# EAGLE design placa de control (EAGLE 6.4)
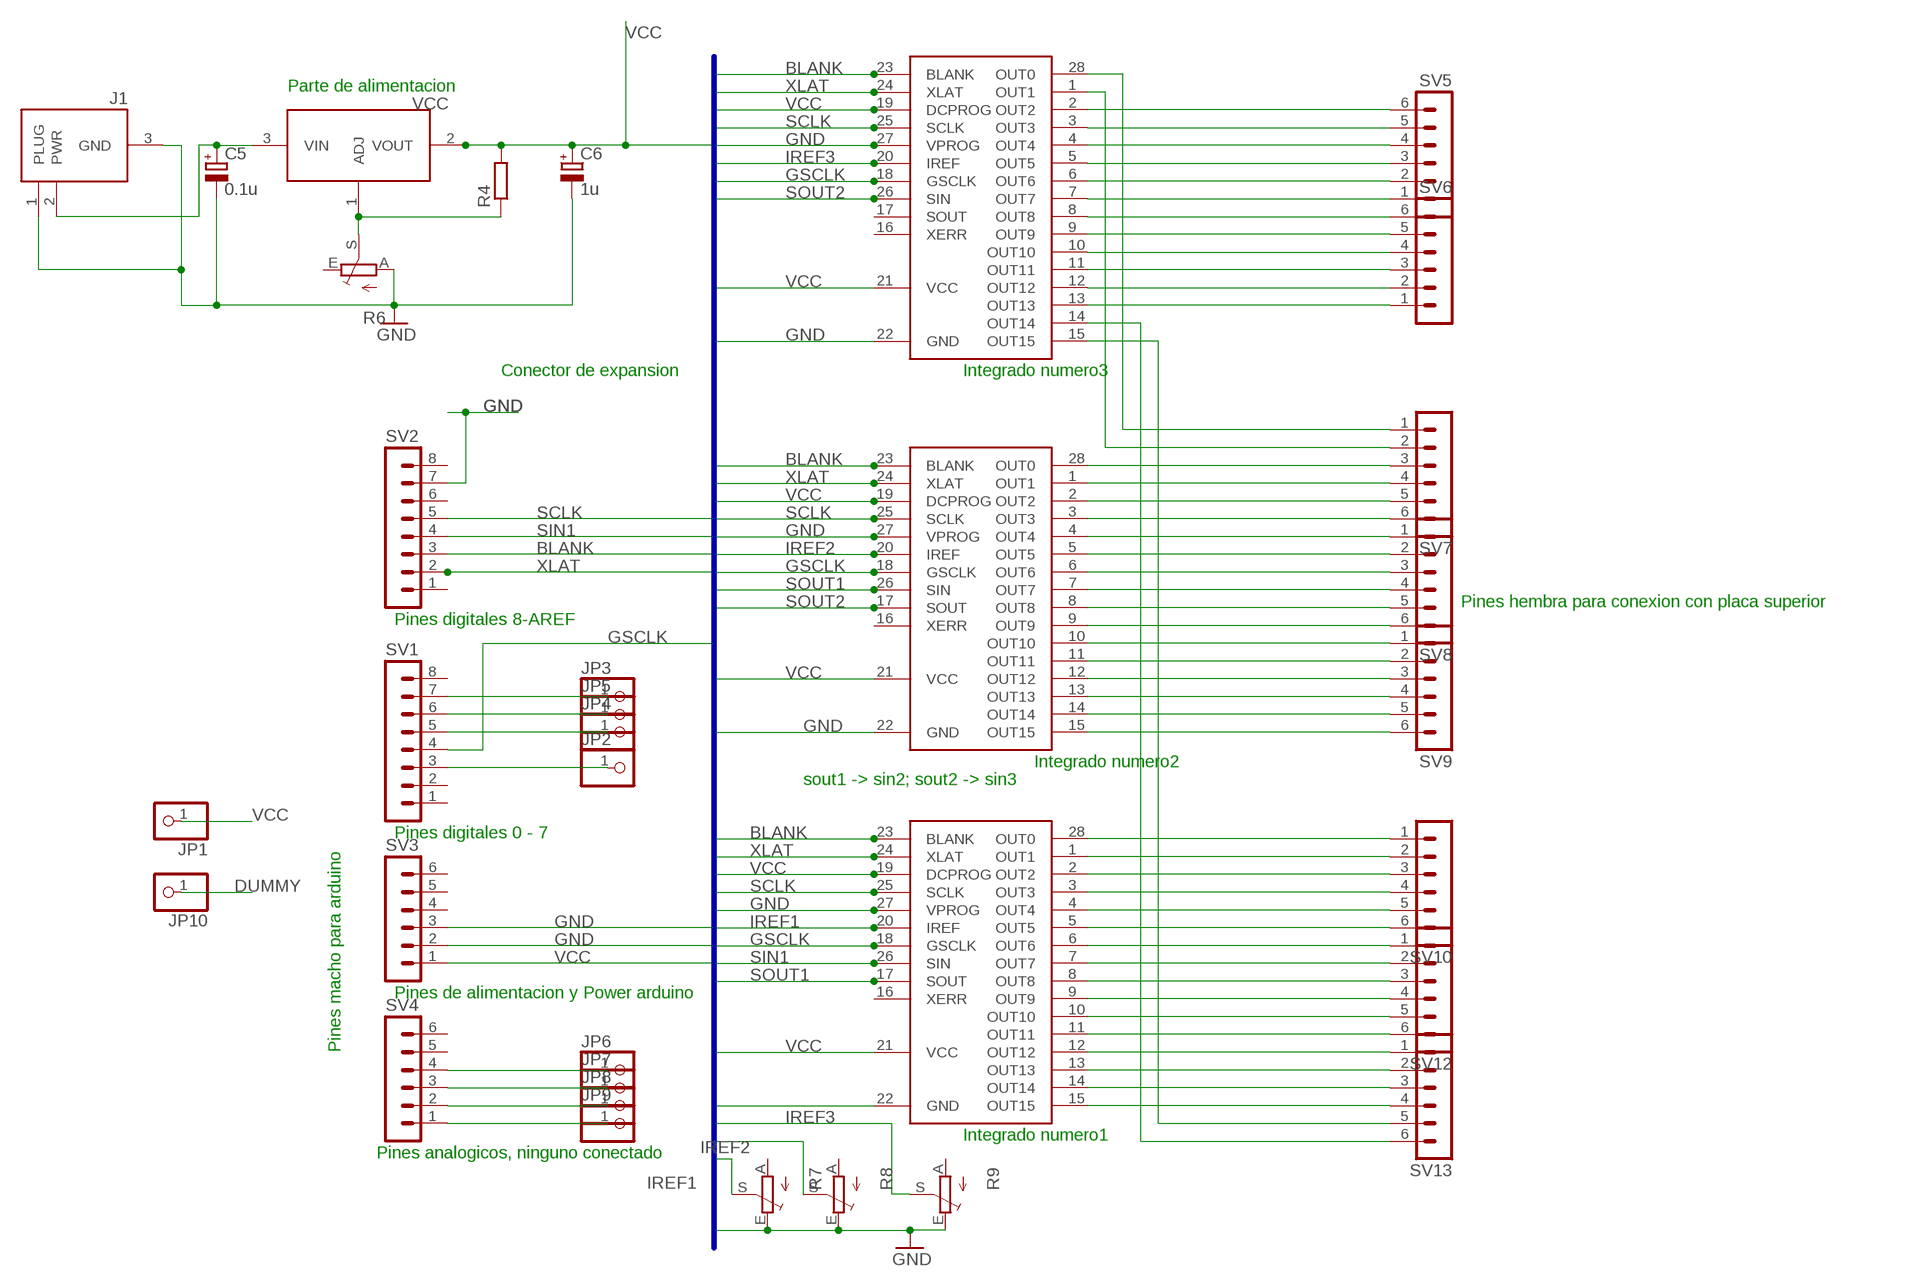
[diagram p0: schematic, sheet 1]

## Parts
C5  0.1u  CPOL-EUE2,5-6E  [E2,5-6E]
C6  1u  CPOL-EUE2,5-6E  [E2,5-6E]
J1  DCJACK-21MM  [DC-21MM]
JP1  PINHD-1X1  [1X01]
JP2  PINHD-1X1  [1X01]
JP3  PINHD-1X1  [1X01]
JP4  PINHD-1X1  [1X01]
JP5  PINHD-1X1  [1X01]
JP6  PINHD-1X1  [1X01]
JP7  PINHD-1X1  [1X01]
JP8  PINHD-1X1  [1X01]
JP9  PINHD-1X1  [1X01]
JP10  PINHD-1X1  [1X01]
R4  R-EU_0204/5  [0204/5]
R6  TRIM_EU-CA9V  [CA9V]
R7  TRIM_EU-CA9V  [CA9V]
R8  TRIM_EU-CA9V  [CA9V]
R9  TRIM_EU-CA9V  [CA9V]
SV1  MA08-1  [MA08-1]
SV2  MA08-1  [MA08-1]
SV3  MA06-1  [MA06-1]
SV4  MA06-1  [MA06-1]
SV5  MA06-1  [MA06-1]
SV6  MA06-1  [MA06-1]
SV7  MA06-1  [MA06-1]
SV8  MA06-1  [MA06-1]
SV9  MA06-1  [MA06-1]
SV10  MA06-1  [MA06-1]
SV12  MA06-1  [MA06-1]
SV13  MA06-1  [MA06-1]
U$1  TLC5940  [DIL28-3]
U$2  TLC5940  [DIL28-3]
U$3  TLC5940  [DIL28-3]
U$4  LM350T  [TO220]

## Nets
ADJ [Vcc]: R4.1 R6.S U$4.1(ADJ)
BLANK: SV2.3 U$1.23(BLANK) U$2.23(BLANK) U$3.23(BLANK)
DUMMY: JP10.1
GND [Vcc]: C5.- C6.- J1.1(PLUG) J1.3(GND) R6.A R7.E R8.E R9.E SV2.7 SV3.2 SV3.3 U$1.22(GND) U$1.27(VPROG) U$2.22(GND) U$2.27(VPROG) U$3.22(GND) U$3.27(VPROG)
GSCLK: SV1.4 U$1.18(GSCLK) U$2.18(GSCLK) U$3.18(GSCLK)
IREF1: R7.S U$2.20(IREF)
IREF2: R8.S U$1.20(IREF)
IREF3: R9.S U$3.20(IREF)
N$2: JP9.1 SV4.1
N$3 [Vcc]: C5.+ J1.2(PWR) U$4.3(VIN)
N$4: JP8.1 SV4.2
N$5: JP7.1 SV4.3
N$6: JP6.1 SV4.4
N$7: JP2.1 SV1.3
N$8: JP3.1 SV1.7
N$9: JP4.1 SV1.5
N$10: JP5.1 SV1.6
N$11: SV10.1 U$2.28(OUT0)
N$12: SV10.2 U$2.1(OUT1)
N$13: SV10.3 U$2.2(OUT2)
N$14: SV10.4 U$2.3(OUT3)
N$15: SV10.5 U$2.4(OUT4)
N$16: SV10.6 U$2.5(OUT5)
N$17: SV12.1 U$2.6(OUT6)
N$18: SV12.2 U$2.7(OUT7)
N$19: SV12.3 U$2.8(OUT8)
N$20: SV12.4 U$2.9(OUT9)
N$21: SV12.5 U$2.10(OUT10)
N$22: SV12.6 U$2.11(OUT11)
N$23: SV13.1 U$2.12(OUT12)
N$24: SV13.2 U$2.13(OUT13)
N$25: SV13.3 U$2.14(OUT14)
N$26: SV13.4 U$2.15(OUT15)
N$27: SV13.5 U$3.15(OUT15)
N$28: SV13.6 U$3.14(OUT14)
N$29: SV9.1 U$1.10(OUT10)
N$30: SV9.2 U$1.11(OUT11)
N$31: SV9.3 U$1.12(OUT12)
N$32: SV9.4 U$1.13(OUT13)
N$33: SV9.5 U$1.14(OUT14)
N$34: SV9.6 U$1.15(OUT15)
N$35: SV8.1 U$1.4(OUT4)
N$36: SV8.2 U$1.5(OUT5)
N$37: SV8.3 U$1.6(OUT6)
N$38: SV8.4 U$1.7(OUT7)
N$39: SV8.5 U$1.8(OUT8)
N$40: SV8.6 U$1.9(OUT9)
N$41: SV7.3 U$1.28(OUT0)
N$42: SV7.4 U$1.1(OUT1)
N$43: SV7.5 U$1.2(OUT2)
N$44: SV7.6 U$1.3(OUT3)
N$45: SV7.1 U$3.28(OUT0)
N$46: SV7.2 U$3.1(OUT1)
N$47: SV5.6 U$3.2(OUT2)
N$48: SV5.5 U$3.3(OUT3)
N$49: SV5.4 U$3.4(OUT4)
N$50: SV5.3 U$3.5(OUT5)
N$51: SV5.2 U$3.6(OUT6)
N$52: SV5.1 U$3.7(OUT7)
N$53: SV6.6 U$3.8(OUT8)
N$54: SV6.5 U$3.9(OUT9)
N$55: SV6.4 U$3.10(OUT10)
N$56: SV6.3 U$3.11(OUT11)
N$57: SV6.2 U$3.12(OUT12)
N$58: SV6.1 U$3.13(OUT13)
SCLK: SV2.5 U$1.25(SCLK) U$2.25(SCLK) U$3.25(SCLK)
SIN1: SV2.4 U$2.26(SIN)
SOUT1: U$1.26(SIN) U$2.17(SOUT)
SOUT2: U$1.17(SOUT) U$3.26(SIN)
VCC [Vcc]: C6.+ JP1.1 R4.2 SV3.1 U$1.19(DCPROG) U$1.21(VCC) U$2.19(DCPROG) U$2.21(VCC) U$3.19(DCPROG) U$3.21(VCC) U$4.2(VOUT)
XLAT: SV2.2 U$1.24(XLAT) U$2.24(XLAT) U$3.24(XLAT)
Unconnected: R6.E R7.A R8.A R9.A SV1.1 SV1.2 SV1.8 SV2.1 SV2.6 SV2.8 SV3.4 SV3.5 SV3.6 SV4.5 SV4.6 U$1.16(XERR) U$2.16(XERR) U$3.16(XERR) U$3.17(SOUT)

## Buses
VCC,GND,BLANK,SIN1,SOUT1,SOUT2,GSCLK,SCLK,XLAT,IREF1,IREF2,IREF3

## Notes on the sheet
- Parte de alimentacion
- Conector de expansion | Integrado numero3
- Pines hembra para conexion con placa superior
- Pines digitales 8-AREF
- Integrado numero2
- sout1 -> sin2; sout2 -> sin3
- Pines digitales 0 - 7
- Pines de alimentacion y Power arduino
- Pines macho para arduino
- Integrado numero1
- Pines analogicos, ninguno conectado

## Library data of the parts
C5 C6 = resistor:CPOL-EU: POLARIZED CAPACITOR, European symbol
J1 = powersupply:DCJACK: 2.1mm DC Power Jack Mouser Part No. 163-5004
JP1-JP10 = pinhead:PINHD-1X1: PIN HEADER
R4 = resistor:R-EU_: RESISTOR, European symbol
R6-R9 = pot:TRIM_EU-: POTENTIOMETER
SV1 SV2 = con-lstb:MA08-1: PIN HEADER; OC_FARNELL: unknown; OC_NEWARK: unknown
SV3-SV10 SV12 SV13 = con-lstb:MA06-1: PIN HEADER; OC_FARNELL: unknown; OC_NEWARK: unknown
U$1-U$3 = tlc5940:TLC5940
U$4 = tlc5940:LM350T

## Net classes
0 Normal: width 0.559 mm, drill 0.559 mm, clearance 0.559 mm
1 Vcc: width 0.762 mm, drill 0.762 mm, clearance 0.762 mm to class 0, clearance 0.762 mm

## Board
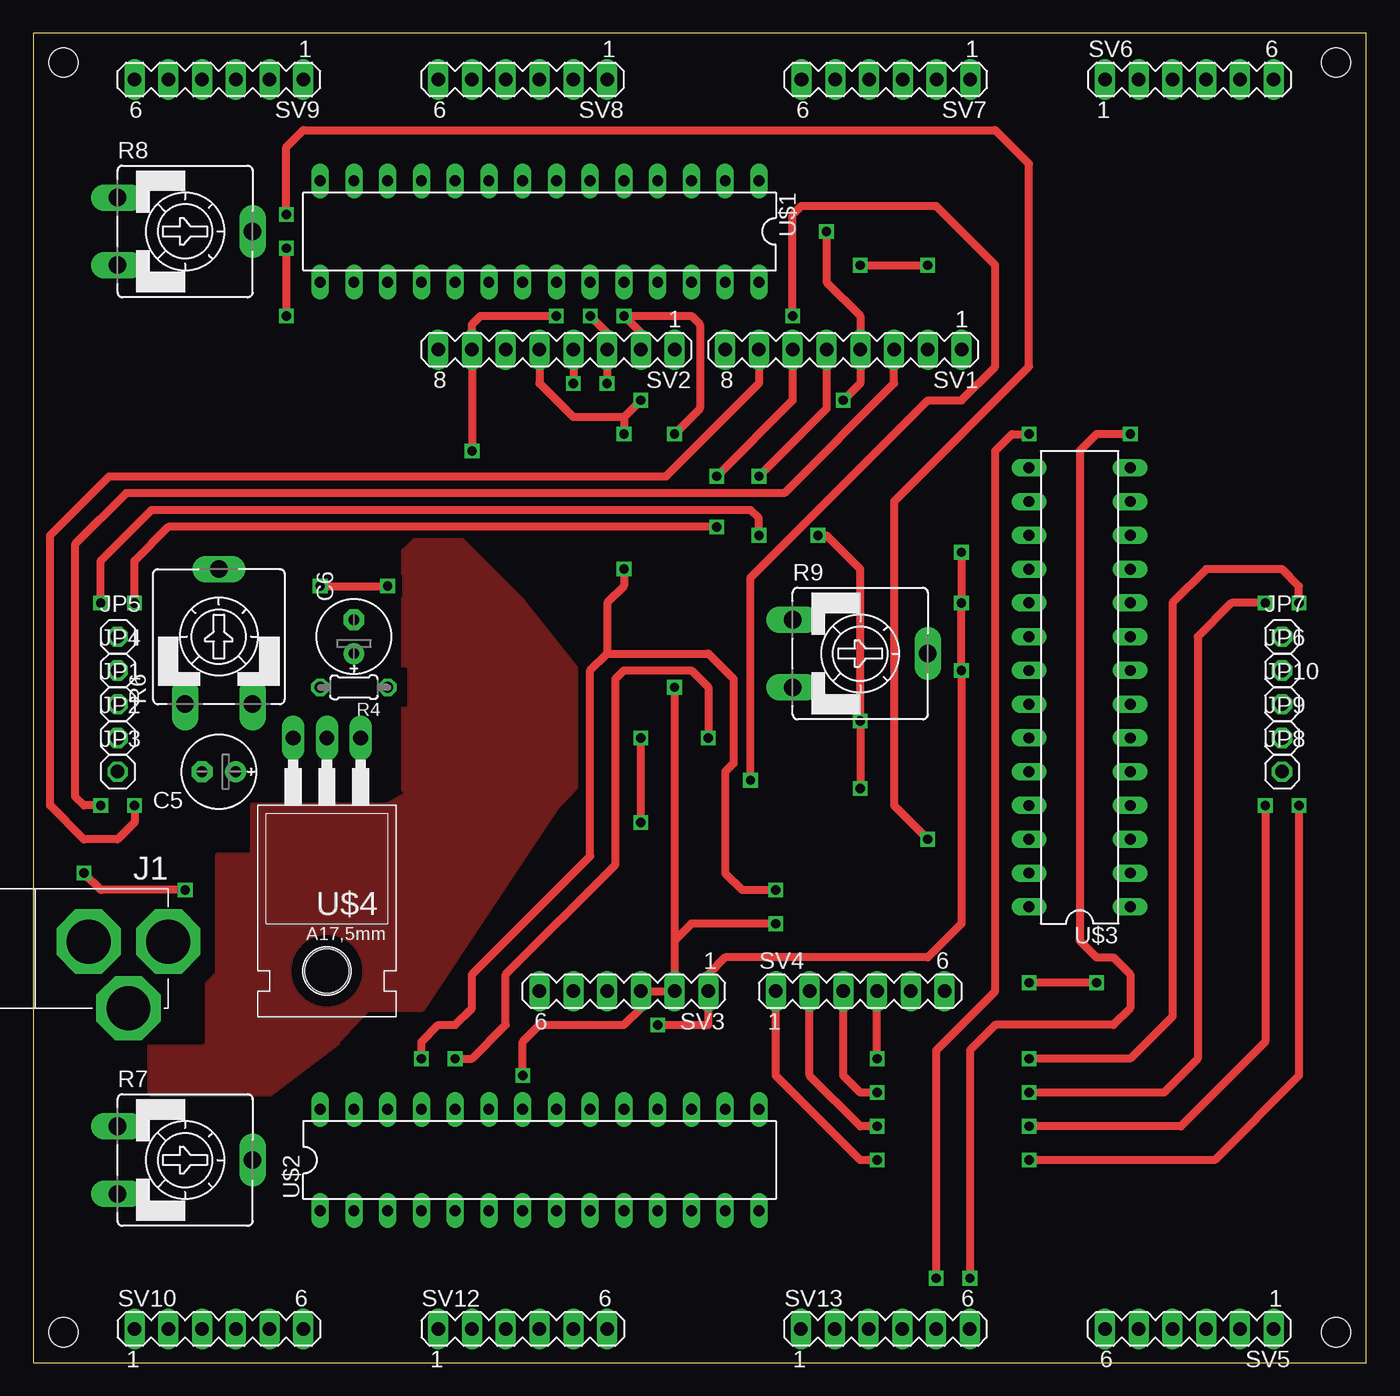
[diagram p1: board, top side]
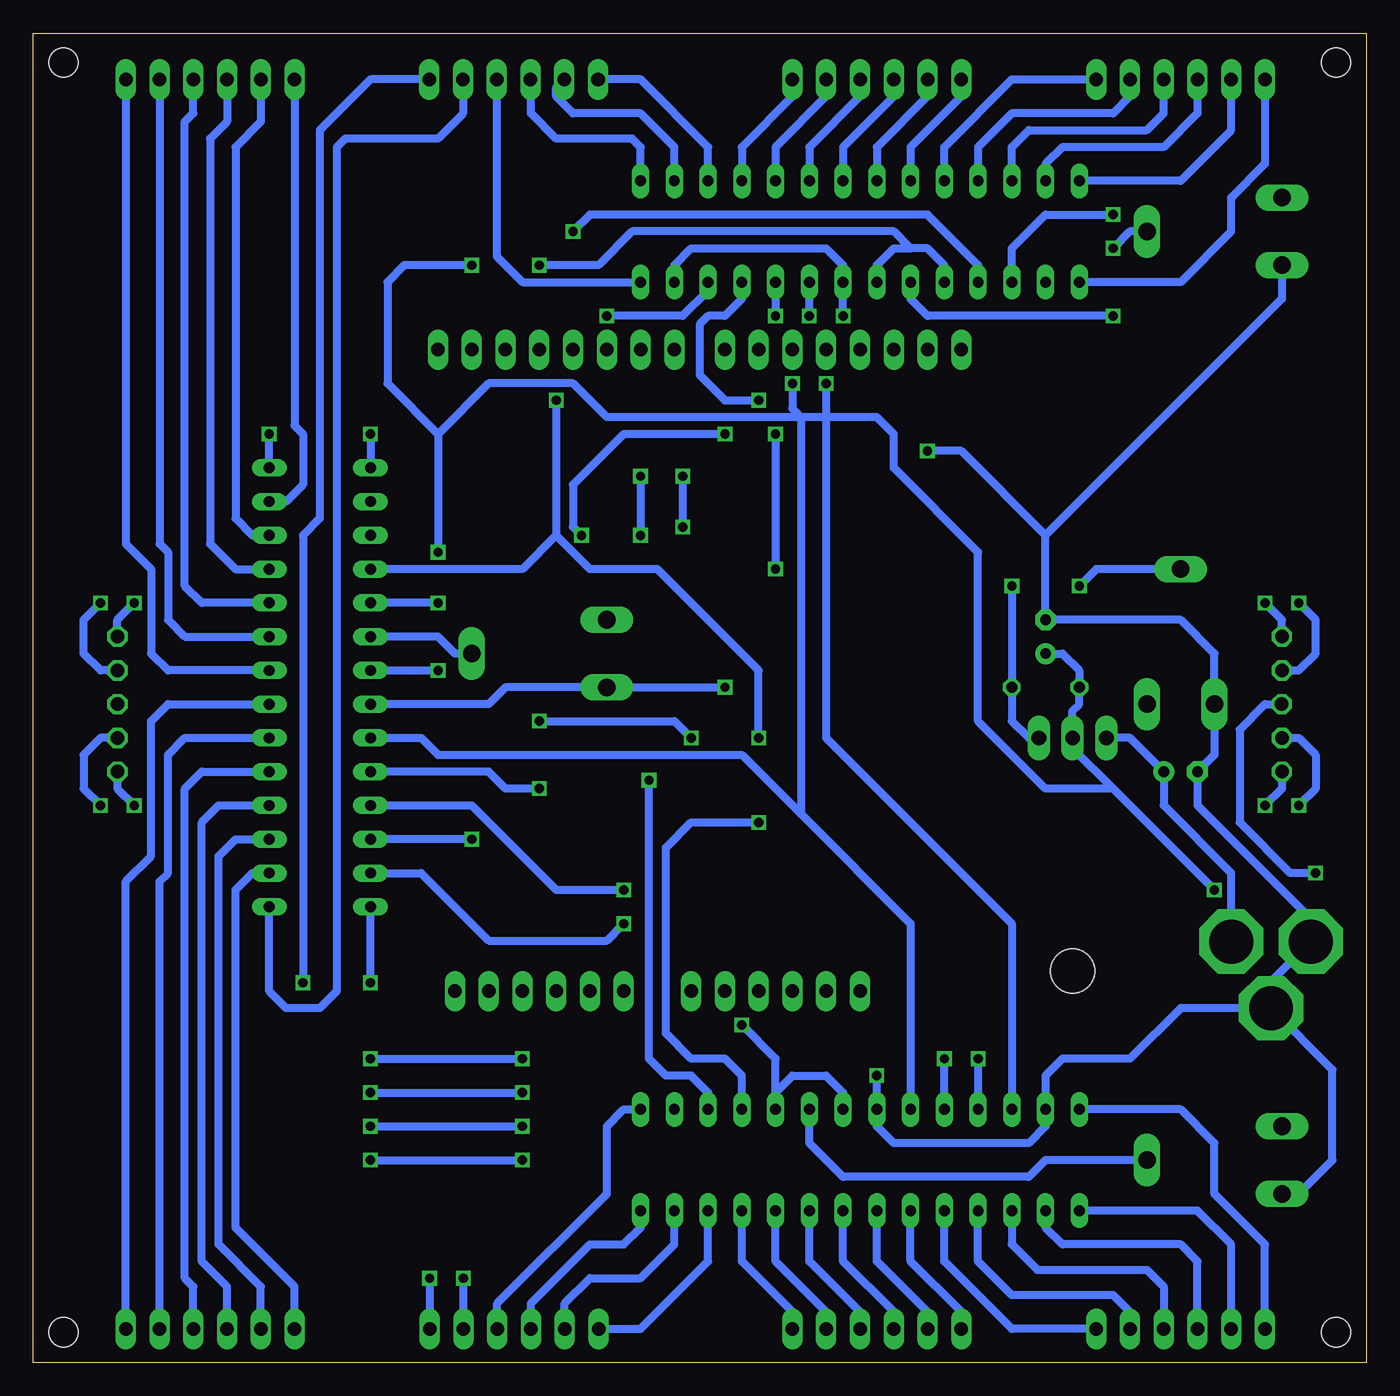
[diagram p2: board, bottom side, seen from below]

Size 100.31 x 100 mm. Coordinates in mm from the lower left corner, seen from the top.
Outline: 0,0 100.31,0 100.31,100 0,100 0,0
Copper layers (1*16): Top 0.035mm / dielectric 1.5mm / Bottom 0.035mm
Design rules "default *": minimum track width 18mil, minimum drill 24mil, track to track 18mil, track to pad 18mil, pad to pad 18mil, via to via 18mil, smd to smd 8mil, copper to edge 40mil, drill to drill 8mil, minimum pad ring 10mil, minimum via ring 8mil, stop-mask expansion 4mil, vias tented up to drill 0mil, thermal gap 10mil
Holes 2.2 mm at 2.29,97.79 98.04,97.79 98.04,2.29 2.29,2.29
tRestrict: area 6.3,95.2 to 21.6,97.8; area 29.2,95.2 to 44.5,97.8; area 57.1,95.2 to 72.4,97.8; area 80,95.2 to 95.2,97.8; area 20.3,87.6 to 55.9,90.2; area 20.3,80 to 55.9,82.5; area 15.2,82.5 to 17.8,87.6; area 3.8,86.4 to 8.9,88.9; area 3.8,81.3 to 8.9,83.8; area 68.6,34.3 to 71.1,69.8; area 76.2,34.3 to 78.7,69.8; area 96.5,54.6 to 99.1,59.7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
bRestrict: area 29.2,74.9 to 49.5,77.5; area 50.8,74.9 to 71.1,77.5; area 36.8,26.7 to 52.1,29.2; area 54.6,26.7 to 69.8,29.2

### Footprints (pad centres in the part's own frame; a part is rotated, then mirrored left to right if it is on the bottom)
E2,5-6E = drill 0.813 pad 1.575: + -1.27,0 | drill 0.813 pad 1.575 octagon: - 1.27,0
DC-21MM = drill 3.302 pad 4.826 octagon: 1 -5.08,-3.353; 2 -0.076,-6.35; 3 -0.076,-0.356
1X01 = drill 1.016 octagon: 1 0,0
0204/5 = drill 0.813 octagon: 1 -2.54,0; 2 2.54,0
CA9V = drill 1.321 long: A -2.54,-5.08; E 2.54,-5.08; S 0,5.08
MA08-1 = drill 1.016 long: 1 -8.89,0; 2 -6.35,0; 3 -3.81,0; 4 -1.27,0; 5 1.27,0; 6 3.81,0; 7 6.35,0; 8 8.89,0
MA06-1 = drill 1.016 long: 1 -6.35,0; 2 -3.81,0; 3 -1.27,0; 4 1.27,0; 5 3.81,0; 6 6.35,0
DIL28-3 = drill 0.813 long: 1 -16.51,-3.81; 2 -13.97,-3.81; 3 -11.43,-3.81; 4 -8.89,-3.81; 5 -6.35,-3.81; 6 -3.81,-3.81; 7 -1.27,-3.81; 8 1.27,-3.81; 9 3.81,-3.81; 10 6.35,-3.81; 11 8.89,-3.81; 12 11.43,-3.81; 13 13.97,-3.81; 14 16.51,-3.81; 15 16.51,3.81; 16 13.97,3.81; 17 11.43,3.81; 18 8.89,3.81; 19 6.35,3.81; 20 3.81,3.81; 21 1.27,3.81; 22 -1.27,3.81; 23 -3.81,3.81; 24 -6.35,3.81; 25 -8.89,3.81; 26 -11.43,3.81; 27 -13.97,3.81; 28 -16.51,3.81
TO220 = drill 1.118 long: 1 -2.54,-6.35; 2 0,-6.35; 3 2.54,-6.35 | hole 3.302: 0,11.176

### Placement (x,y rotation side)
C5  13.97,44.45 180 top
C6  24.13,54.61 90 top
J1  3.81,31.75 90 top
JP1  6.36,49.53 0 top
JP2  6.35,46.99 0 top
JP3  6.35,44.45 0 top
JP4  6.35,52.07 0 top
JP5  6.35,54.61 0 top
JP6  93.98,52.07 0 top
JP7  93.98,54.61 0 top
JP8  93.98,44.45 0 top
JP9  93.98,46.99 0 top
JP10  93.98,49.53 0 top
R4  24.13,50.8 180 top
R6  13.97,54.61 0 top
R7  11.43,15.24 270 top
R8  11.43,85.09 270 top
R9  62.23,53.34 270 top
SV1  60.96,76.2 180 top
SV2  39.37,76.2 180 top
SV3  44.45,27.94 180 top
SV4  62.23,27.94 0 top
SV5  87,2.54 180 top
SV6  87,96.52 0 top
SV7  64.16,96.52 180 top
SV8  36.83,96.52 180 top
SV9  13.97,96.52 180 top
SV10  13.97,2.54 0 top
SV12  36.83,2.54 0 top
SV13  64.12,2.54 0 top
U$1  38.1,85.09 180 top
U$2  38.1,15.24 0 top
U$3  78.74,50.8 90 top
U$4  22.1,40.64 180 top

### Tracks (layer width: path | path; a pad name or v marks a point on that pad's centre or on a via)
ADJ  (via drill 0.7)
  Top 0.61: v21.59,58.42 v26.67,58.42
  Bottom 0.61: v26.67,58.42 R4.1 26.67,48.26 25.4,46.99 U$4.1 | R6.S 20.32,59.69 v21.59,58.42
BLANK  (via drill 0.7)
  Top 0.61: v41.91,78.74 43.18,77.47 SV2.3 v43.18,73.66
  Bottom 0.61: v41.91,78.74 U$1.23 | 42.55,41.27 46.99,45.72 69.85,45.72 71.12,46.99 U$3.23 | 42.55,41.27 34.29,33.02 U$2.23 | v43.18,73.66 43.18,71.75 42.55,71.12 42.55,41.27
E
  pour Top: 41.91,50.8 41.91,44.45 22.86,24.13 16.51,24.13 16.51,41.91 26.67,41.91
  pour Top: 41.91,50.8 27.94,38.1 30.48,45.72 31.75,50.8 33.02,52.07 36.83,57.15
  pour Top: 36.83,57.15 30.48,63.5 27.94,60.96 34.29,54.61
  pour Top: 16.51,38.1 13.97,38.1 13.97,29.21 8.89,24.13 8.89,20.32 17.78,20.32 22.86,24.13 16.51,24.13
  pour Top: 27.94,60.96 27.94,43.18 34.29,43.18 34.29,58.42 30.48,58.42 30.48,60.96
GND  (via drill 0.7)
  Top 0.61: v39.37,78.74 33.66,78.74 33.02,78.11 SV2.7 v33.02,68.58 | v48.26,50.8 48.26,31.75 | 48.26,31.75 SV3.2 SV3.3 45.72,26.67 44.45,25.4 38.1,25.4 36.83,24.13 v36.83,21.59 | v55.88,33.02 49.53,33.02 48.26,31.75
  Bottom 0.61: R7.E 5.08,12.7 2.54,15.24 2.54,22.05 J1.1 | J1.1 7.16,28.68 J1.3 4.17,33.38 12.7,41.91 C5.- 11.43,45.72 R6.A 11.43,53.34 13.97,55.88 C6.- 24.13,62.23 | J1.1 13.97,26.67 17.78,22.86 22.86,22.86 24.13,21.59 U$2.27 24.13,17.78 25.4,16.51 35.56,16.51 36.83,17.78 U$2.22 v36.83,21.59 | U$1.27 52.07,82.55 50.8,83.82 40.64,83.82 39.37,82.55 U$1.22 v39.37,78.74 | U$3.22 66.04,49.53 64.77,50.8 R9.E v48.26,50.8 | U$3.27 71.12,36.83 66.04,31.75 57.15,31.75 v55.88,33.02 | 24.13,62.23 30.48,68.58 v33.02,68.58 | R8.E 6.35,80.01 24.13,62.23
GSCLK  (via drill 0.7)
  Top 0.61: v59.69,85.09 59.69,81.28 62.23,78.74 SV1.4 62.23,73.66 v60.96,72.39 | v45.72,40.64 v45.72,46.99
  Bottom 0.61: U$1.18 29.21,82.55 33.02,86.36 58.42,86.36 v59.69,85.09 | v60.96,72.39 60.96,62.23 | 60.96,62.23 63.5,59.69 U$3.18 | U$2.18 46.99,21.59 48.26,22.86 50.8,22.86 52.7,24.77 52.7,38.73 50.8,40.64 v45.72,40.64 | v45.72,46.99 45.72,52.07 53.34,59.69 58.42,59.69 60.96,62.23
IREF1
  Bottom 0.61: R7.S 24.13,15.24 25.4,13.97 39.37,13.97 41.91,16.51 U$2.20
IREF2  (via drill 0.7)
  Top 0.61: v19.05,83.82 v19.05,78.74
  Bottom 0.61: v19.05,78.74 33.02,78.74 34.29,80.01 U$1.20 | R8.S 17.78,85.09 v19.05,83.82
IREF3
  Bottom 0.61: R9.S 68.58,53.34 69.85,54.61 U$3.20
N$1
  pour Top: 25.4,26.67 29.21,26.67 39.37,41.91
N$2  (via drill 0.7)
  Top 0.61: v74.93,15.24 88.9,15.24 95.25,21.59 v95.25,41.91 | v63.5,15.24 62.23,15.24 55.88,21.59 SV4.1
  Bottom 0.61: v74.93,15.24 v63.5,15.24 | JP9.1 95.25,46.99 96.52,45.72 96.52,43.18 v95.25,41.91
N$3
  Bottom 0.61: J1.2 10.16,36.83 15.24,41.91 C5.+ 17.78,46.99 U$4.3
N$4  (via drill 0.7)
  Top 0.61: v74.93,17.78 86.36,17.78 92.71,24.13 v92.71,41.91 | v63.5,17.78 62.23,17.78 58.42,21.59 SV4.2
  Bottom 0.61: v74.93,17.78 v63.5,17.78 | JP8.1 93.98,43.18 v92.71,41.91
N$5  (via drill 0.7)
  Top 0.61: v74.93,20.32 85.09,20.32 87.63,22.86 87.63,54.61 90.17,57.15 v92.71,57.15 | v63.5,20.32 62.23,20.32 60.96,21.59 SV4.3
  Bottom 0.61: v74.93,20.32 v63.5,20.32 | JP7.1 93.98,55.88 v92.71,57.15
N$6  (via drill 0.7)
  Top 0.61: v74.93,22.86 82.55,22.86 85.72,26.04 85.72,57.15 88.27,59.69 93.98,59.69 95.25,58.42 v95.25,57.15 | v63.5,22.86 SV4.4
  Bottom 0.61: v74.93,22.86 v63.5,22.86 | JP6.1 95.25,52.07 96.52,53.34 96.52,55.88 v95.25,57.15
N$7  (via drill 0.7)
  Top 0.61: SV1.3 64.77,73.66 56.52,65.41 6.99,65.41 3.17,61.59 3.17,42.55 3.81,41.91 v5.08,41.91
  Bottom 0.61: JP2.1 5.08,46.99 3.81,45.72 3.81,43.18 v5.08,41.91
N$8  (via drill 0.7)
  Top 0.61: SV1.7 54.61,73.66 47.62,66.67 5.71,66.67 1.27,62.23 1.27,41.91 3.81,39.37 6.35,39.37 7.62,40.64 v7.62,41.91
  Bottom 0.61: JP3.1 6.35,43.18 v7.62,41.91
N$9  (via drill 0.7)
  Top 0.61: SV1.5 59.69,71.75 v54.61,66.67 | v54.61,62.23 54.61,63.5 53.98,64.14 8.89,64.14 5.08,60.33 v5.08,57.15
  Bottom 0.61: v54.61,66.67 v54.61,62.23 | JP4.1 5.08,52.07 3.81,53.34 3.81,55.88 v5.08,57.15
N$10  (via drill 0.7)
  Top 0.61: SV1.6 57.15,72.39 v51.44,66.67 | v51.44,62.87 10.16,62.87 7.62,60.33 v7.62,57.15
  Bottom 0.61: v51.44,66.67 v51.44,62.87 | JP5.1 6.35,55.88 v7.62,57.15
N$11
  Bottom 0.61: SV10.1 7.62,8.89 11.43,12.7 11.43,16.51 13.97,19.05 U$2.28
N$12
  Bottom 0.61: SV10.2 10.16,8.89 12.7,11.43 U$2.1
N$13
  Bottom 0.61: SV10.3 12.7,7.62 13.97,8.89 22.86,8.89 24.13,10.16 U$2.2
N$14
  Bottom 0.61: U$2.3 26.67,8.89 24.77,6.99 16.51,6.99 15.24,5.71 SV10.4
N$15
  Bottom 0.61: SV10.5 17.78,3.81 19.05,5.08 26.67,5.08 29.21,7.62 U$2.4
N$16
  Bottom 0.61: SV10.6 26.67,2.54 31.75,7.62 U$2.5
N$17
  Bottom 0.61: SV12.1 30.48,3.81 34.29,7.62 U$2.6
N$18
  Bottom 0.61: SV12.2 33.02,3.81 36.83,7.62 U$2.7
N$19
  Bottom 0.61: SV12.3 35.56,3.81 39.37,7.62 U$2.8
N$20
  Bottom 0.61: SV12.4 38.1,3.81 41.91,7.62 U$2.9
N$21
  Bottom 0.61: SV12.5 40.64,3.81 44.45,7.62 U$2.10
N$22
  Bottom 0.61: SV12.6 43.18,3.81 46.99,7.62 U$2.11
N$23
  Bottom 0.61: SV13.1 54.61,2.54 49.53,7.62 U$2.12
N$24
  Bottom 0.61: SV13.2 60.31,4.46 58.42,6.35 54.61,6.35 52.07,8.89 U$2.13
N$25
  Bottom 0.61: SV13.3 62.85,4.46 58.42,8.89 55.88,8.89 54.61,10.16 U$2.14
N$26
  Bottom 0.61: SV13.4 65.39,4.46 57.15,12.7 57.15,17.78 55.88,19.05 U$2.15
N$27  (via drill 0.7)
  Top 0.61: v67.94,6.35 67.94,23.5 72.39,27.94 72.39,68.58 73.66,69.85 v74.93,69.85
  Bottom 0.61: SV13.5 67.93,6.34 v67.94,6.35 | v74.93,69.85 U$3.15
N$28  (via drill 0.7)
  Top 0.61: v82.55,69.85 80.01,69.85 78.74,68.58 78.74,31.75 80.01,30.48 81.28,30.48 82.55,29.21 82.55,26.67 81.28,25.4 72.39,25.4 70.48,23.5 v70.48,6.35
  Bottom 0.61: U$3.14 v82.55,69.85 | v70.48,6.35 70.48,2.55 SV13.6
N$29
  Bottom 0.61: U$1.10 31.75,91.44 26.67,96.52 SV9.1
N$30
  Bottom 0.61: SV9.2 17.78,95.25 19.05,93.98 26.67,93.98 29.21,91.44 U$1.11
N$31
  Bottom 0.61: U$1.12 26.67,91.44 25.4,92.71 16.51,92.71 15.24,93.98 SV9.3
N$32
  Bottom 0.61: SV9.4 12.7,93.98 15.24,91.44 22.86,91.44 24.13,90.17 U$1.13
N$33
  Bottom 0.61: SV9.5 10.16,92.71 13.97,88.9 U$1.14
N$34
  Bottom 0.61: SV9.6 7.62,90.17 10.16,87.63 10.16,85.09 13.97,81.28 U$1.15
N$35
  Bottom 0.61: SV8.1 43.18,95.25 46.99,91.44 U$1.4
N$36
  Bottom 0.61: SV8.2 40.64,95.25 44.45,91.44 U$1.5
N$37
  Bottom 0.61: SV8.3 38.1,95.25 41.91,91.44 U$1.6
N$38
  Bottom 0.61: SV8.4 35.56,95.25 39.37,91.44 U$1.7
N$39
  Bottom 0.61: SV8.5 33.02,95.25 36.83,91.44 U$1.8
N$40
  Bottom 0.61: SV8.6 30.48,95.25 34.29,91.44 U$1.9
N$41
  Bottom 0.61: SV7.3 65.43,83.21 63.5,81.28 U$1.28
N$42
  Bottom 0.61: U$1.1 54.61,91.44 55.24,92.08 60.96,92.08 62.87,93.98 62.87,96.5 SV7.4
N$43
  Bottom 0.61: U$1.2 52.07,91.44 54.61,93.98 59.69,93.98 60.96,95.25 60.96,95.91 SV7.5
N$44
  Bottom 0.61: U$1.3 49.53,91.44 54.61,96.52 SV7.6
N$45  (via drill 0.7)
  Top 0.61: v80.01,28.57 v74.93,28.57
  Bottom 0.61: SV7.1 74.93,96.52 78.74,92.71 78.74,63.5 80.01,62.23 v80.01,28.57 | v74.93,28.57 U$3.28
N$46
  Bottom 0.61: SV7.2 67.97,93.96 69.85,92.08 76.83,92.08 77.47,91.44 77.47,27.94 78.74,26.67 81.28,26.67 82.55,27.94 U$3.1
N$47
  Bottom 0.61: SV5.6 80.64,5.71 85.09,10.16 85.09,35.56 83.82,36.83 U$3.2
N$48
  Bottom 0.61: SV5.5 83.19,5.71 86.36,8.89 86.36,38.1 85.09,39.37 U$3.3
N$49
  Bottom 0.61: SV5.4 85.72,5.71 87.63,7.62 87.63,40.64 86.36,41.91 U$3.4
N$50
  Bottom 0.61: SV5.3 88.27,5.71 88.9,6.35 88.9,43.18 87.63,44.45 U$3.5
N$51
  Bottom 0.61: SV5.2 90.81,36.2 90.17,36.83 90.17,45.72 88.9,46.99 U$3.6
N$52
  Bottom 0.61: SV5.1 93.34,36.2 91.44,38.1 91.44,48.26 90.17,49.53 U$3.7
N$53
  Bottom 0.61: SV6.6 93.34,61.59 91.44,59.69 91.44,53.34 90.17,52.07 U$3.8
N$54
  Bottom 0.61: SV6.5 90.81,61.59 90.17,60.96 90.17,55.88 88.9,54.61 U$3.9
N$55
  Bottom 0.61: U$3.10 87.63,57.15 88.9,58.42 88.9,93.34 88.27,93.98 SV6.4
N$56
  Bottom 0.61: SV6.3 85.72,93.34 87,92.08 87,61.59 85.09,59.69 U$3.11
N$57
  Bottom 0.61: SV6.2 83.19,93.34 85.09,91.44 85.09,63.5 83.82,62.23 U$3.12
N$58
  Bottom 0.61: U$3.13 81.28,64.77 80.01,66.04 80.01,69.85 80.64,70.48 SV6.1
SCLK  (via drill 0.7)
  Top 0.61: SV2.5 38.1,73.66 40.64,71.12 44.45,71.12 | v45.72,72.39 44.45,71.12 | v29.21,22.86 29.21,24.13 30.48,25.4 31.75,25.4 33.02,26.67 33.02,29.21 41.91,38.1 41.91,52.07 43.18,53.34 | 43.18,53.34 50.8,53.34 52.7,51.44 52.7,45.09 52.07,44.45 52.07,36.83 53.34,35.56 v55.88,35.56 | 44.45,71.12 v44.45,69.85 | v44.45,59.69 44.45,58.42 43.18,57.15 43.18,53.34
  Bottom 0.61: U$1.25 46.99,80.01 48.26,78.74 49.53,78.74 50.16,78.11 50.16,74.3 48.26,72.39 v45.72,72.39 | U$3.25 67.31,41.91 60.96,35.56 v55.88,35.56 | v29.21,22.86 U$2.25 | v44.45,69.85 v44.45,59.69
SIN1  (via drill 0.7)
  Top 0.61: SV2.4 v40.64,73.66
  Bottom 0.61: v40.64,73.66 40.64,46.99 26.67,33.02 U$2.26
SOUT1  (via drill 0.7)
  Top 0.61: v53.98,43.81 53.98,59.05 67.31,72.39 69.85,72.39 72.39,74.93 72.39,82.55 67.94,87 57.78,87 57.15,86.36 v57.15,78.74
  Bottom 0.61: U$2.17 49.53,20.32 50.8,21.59 52.7,21.59 53.98,22.86 v53.98,43.81 | U$1.26 49.53,80.64 51.44,78.74 v57.15,78.74
SOUT2  (via drill 0.7)
  Top 0.61: v19.05,86.36 19.05,91.44 20.32,92.71 72.39,92.71 74.93,90.17 74.93,74.93 64.77,64.77 64.77,41.91 v67.31,39.37
  Bottom 0.61: U$1.17 26.67,83.82 24.13,86.36 v19.05,86.36 | v67.31,39.37 U$3.26
VCC  (via drill 0.7)
  Top 0.61: v62.23,82.55 v67.31,82.55 | v69.85,60.96 v69.85,57.15 v69.85,52.07 69.85,33.02 67.31,30.48 52.07,30.48 50.8,29.21 SV3.1 50.8,25.4 v46.99,25.4 | v11.43,35.56 5.08,35.56 v3.81,36.83
  Bottom 0.61: U$1.19 31.75,82.55 33.02,83.82 34.29,83.82 | 34.29,83.82 35.56,85.09 55.24,85.09 57.78,82.55 v62.23,82.55 | U$1.21 36.83,82.55 35.56,83.82 34.29,83.82 | v67.31,82.55 72.39,82.55 73.66,81.28 73.66,73.66 69.85,69.85 | 69.85,69.85 v69.85,60.96 | v69.85,57.15 U$3.19 | U$3.21 v69.85,52.07 | U$2.21 39.37,20.32 40.64,21.59 43.18,21.59 44.45,20.32 U$2.19 44.45,22.86 v46.99,25.4 | 19.05,43.18 22.1,46.23 U$4.2 22.1,49.02 21.59,49.53 R4.2 21.59,52.07 22.86,53.34 C6.+ | 19.05,43.18 24.13,43.18 29.21,48.26 29.21,60.96 35.56,67.31 35.56,69.85 36.83,71.12 57.15,71.12 59.69,73.66 66.04,73.66 69.85,69.85 | 19.05,43.18 v11.43,35.56 | v3.81,36.83 5.71,36.83 9.53,40.64 9.53,47.62 7.62,49.53 JP1.1
XLAT  (via drill 0.7)
  Top 0.61: v48.26,69.85 50.16,71.75 50.16,78.11 49.53,78.74 v44.45,78.74 45.72,77.47 SV2.2 | v59.05,62.23 59.69,62.23 62.23,59.69 v62.23,48.26 v62.23,43.18 | v31.75,22.86 33.02,22.86 35.56,25.4 35.56,29.21 43.81,37.47 43.81,51.44 44.45,52.07 49.53,52.07 50.8,50.8 v50.8,46.99
  Bottom 0.61: U$1.24 v44.45,78.74 | v48.26,69.85 55.88,69.85 59.69,66.04 59.69,62.87 v59.05,62.23 | U$2.24 v31.75,22.86 | v62.23,43.18 64.77,43.18 66.04,44.45 U$3.24 | v62.23,48.26 52.07,48.26 v50.8,46.99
